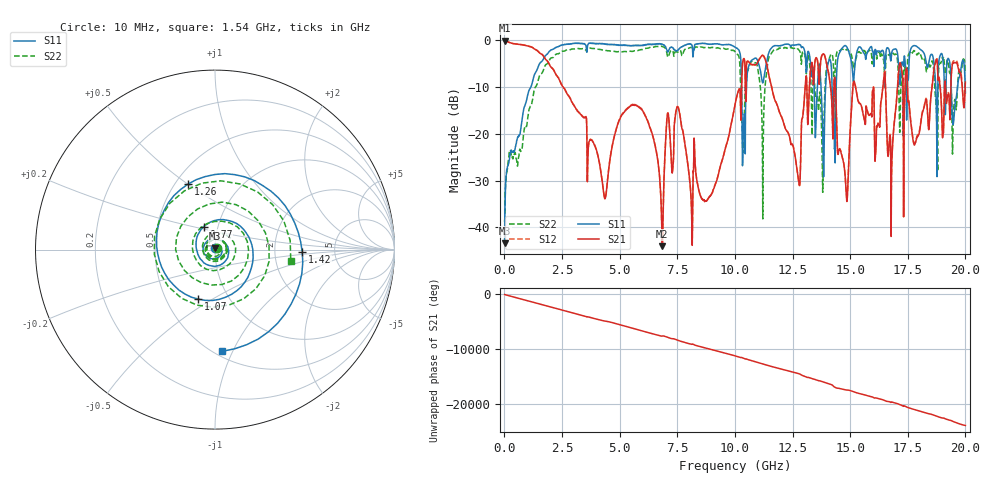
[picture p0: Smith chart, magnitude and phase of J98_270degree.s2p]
!Keysight Technologies,N5222A,MY51421036,A.10.65.16
!Date: Friday, March 31, 2023 14:41:30
!Correction: S11(Full 2 Port(1,2))
!S21(Full 2 Port(1,2))
!S12(Full 2 Port(1,2))
!S22(Full 2 Port(1,2))
!S2P File: Measurements: S11, S21, S12, S22:
# Hz S  dB  R 50
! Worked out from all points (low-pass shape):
!   2000 points, 10 MHz to 20 GHz, reference 50 ohm
!   highest |S21| = -0.07 dB at 20 MHz (marker M1); lowest = -44.0 dB at 6.85 GHz (marker M2)
!   |S21| within 3 dB of the highest: start of sweep to 1.644 GHz; 13.79 GHz to 13.88 GHz (81.15 MHz wide, 0.587 % of centre)
!   lowest |S11| = -43.4 dB at 10 MHz (marker M3), VSWR 1.01, Z = 50.1 + j0.667 ohm
!   |S11| at or under -10 dB: start of sweep to 1.15 GHz; 10.29 GHz to 10.5 GHz (211.7 MHz wide, 2.04 % of centre); 19.39 GHz to 19.66 GHz (271.8 MHz wide, 1.39 % of centre)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
!   |S22| runs from -38.8 to -1.3 dB; largest |S21 - S12| = 0.037
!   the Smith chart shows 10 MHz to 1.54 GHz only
!   S11 on the Smith chart (normalised r, x): 10 MHz: 1.00, +0.01; 770 MHz: 0.85, +0.22; 1.07 GHz: 0.72, -0.43; 1.26 GHz: 0.58, +0.50; 1.42 GHz: 2.89, -0.10; 1.54 GHz: 0.55, -0.91
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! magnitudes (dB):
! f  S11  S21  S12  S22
! 10 MHz  -43.4  -0.1  0.0  -38.8
! 20 MHz  -36.8  -0.1  -0.1  -37.7
! 770 MHz  -16.9  -1.0  -1.0  -23.2
! 1.07 GHz  -10.7  -1.3  -1.3  -14.8
! 1.26 GHz  -8.1  -1.7  -1.7  -11.4
! 1.42 GHz  -6.3  -2.2  -2.2  -9.4
! 1.54 GHz  -4.9  -2.8  -2.7  -7.4
! 3.35 GHz  -0.7  -16.1  -16.0  -1.8
! 6.68 GHz  -0.8  -26.6  -26.5  -1.4
! 6.85 GHz  -0.8  -44.0  -44.0  -1.3
! 7.5 GHz  -2.2  -14.2  -14.2  -2.6
! 8.72 GHz  -0.7  -34.3  -34.4  -1.5
! 10.01 GHz  -1.5  -13.7  -13.7  -2.5
! 11.25 GHz  -8.3  -3.4  -3.4  -16.2
! 12.75 GHz  -0.9  -29.6  -29.6  -1.9
! 13.34 GHz  -7.8  -4.8  -4.7  -19.3
! 14.82 GHz  -1.2  -32.0  -31.9  -2.1
! 15.19 GHz  -6.2  -9.0  -8.9  -5.4
! 16.67 GHz  -1.8  -23.9  -23.7  -3.1
! 17.18 GHz  -8.5  -4.9  -4.7  -13.2
! 17.81 GHz  -1.1  -22.2  -22.0  -2.4
! 20 GHz  -11.2  -8.9  -8.5  -7.0
